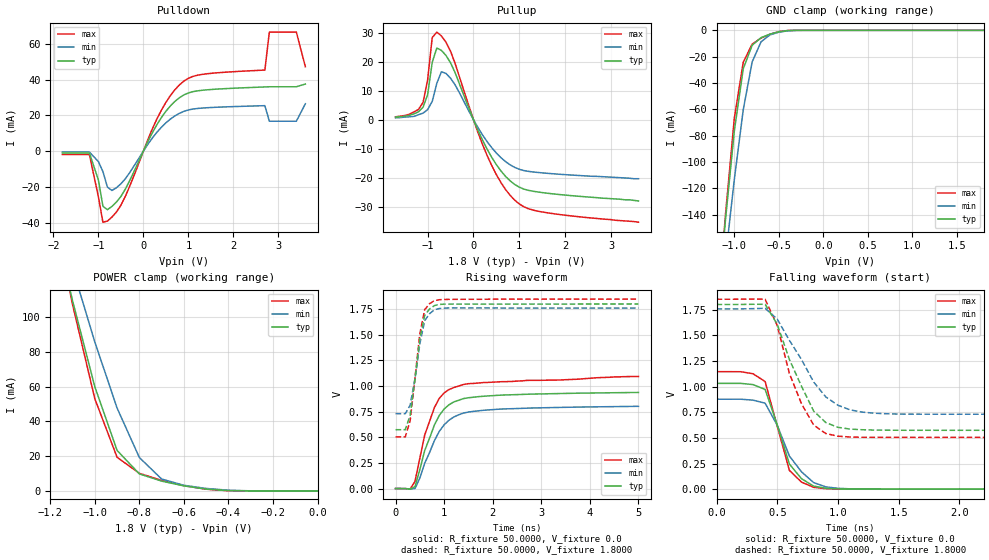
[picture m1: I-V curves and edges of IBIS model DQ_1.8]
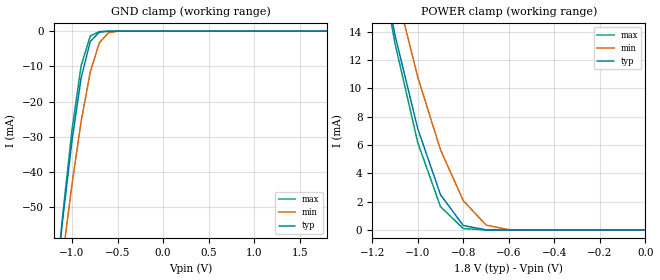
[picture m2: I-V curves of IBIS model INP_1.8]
|*** ISSI Synchronous Sram IBIS Model ***
[IBIS ver]	3.2
[File name]	is61vvps204836b100tq.ibs
[File Rev]	1.0
[Date]	May 13,2013
[Notes]
|--- Version History --------------------------------
|1.0: prelimiary
[Disclaimer]	This information is for modeling purpose only
		and is not guaranteed
[Copyright]	INTEGRATED SILICON SOLUTION, INC. 2011
[Component]	IS61VVPS204836B_100TQ
[Manufacturer]	ISSI
[Package]
| variable   typ   min   max
R_pkg		105.88m			21.330m			174.58m
L_pkg		1.8700nH		0.5900nH		2.5200nH
C_pkg		0.2100pF		0.0600pF		0.2800pF
[Pin]  signal_name   model_name   R_pin   L_pin   C_pin
100   A   INP_1.8
99   A   INP_1.8
98   CEB   INP_1.8
97   CE2   INP_1.8
96   NC   NC
95   NC   NC
94   BWbB   INP_1.8
93   BWaB   INP_1.8
92   CE2B   INP_1.8
91   VDD   POWER
90   VSS   GND
89   CLK   INP_1.8
88   GWB   INP_1.8
87   BWEB   INP_1.8
86   OEB   INP_1.8
85   ADSCB   INP_1.8
84   ADSPB   INP_1.8
83   ADVB   INP_1.8
82   A   INP_1.8
81   A   INP_1.8
80   DQPb   DQ_1.8
79   DQb   DQ_1.8
78   DQb   DQ_1.8
77   VDDQ   POWER
76   VSS   GND
75   DQb   DQ_1.8
74   DQb   DQ_1.8
73   DQb   DQ_1.8
72   DQb   DQ_1.8
71   VSS   GND
70   VDDQ   POWER
69   DQb   DQ_1.8
68   DQb   DQ_1.8
67   VSS   GND
66   NC   NC
65   VDD   POWER
64   ZZ   INP_1.8
63   DQa   DQ_1.8
62   DQa   DQ_1.8
61   VDDQ   POWER
60   VSS   GND
59   DQa   DQ_1.8
58   DQa   DQ_1.8
57   DQa   DQ_1.8
56   DQa   DQ_1.8
55   VSS   GND
54   VDDQ   POWER
53   DQa   DQ_1.8
52   DQa   DQ_1.8
51   DQPa   DQ_1.8
50   A   INP_1.8
49   A   INP_1.8
48   A   INP_1.8
47   A   INP_1.8
46   A   INP_1.8
45   A   INP_1.8
44   A   INP_1.8
43   A   INP_1.8
42   A   INP_1.8
41   VDD   POWER
40   VSS   GND
39   A   INP_1.8
38   A   INP_1.8
37   A0   INP_1.8
36   A1   INP_1.8
35   A   INP_1.8
34   A   INP_1.8
33   A   INP_1.8
32   A   INP_1.8
31   MODE   INP_1.8
30   DQPd   DQ_1.8
29   DQd   DQ_1.8
28   DQd   DQ_1.8
27   VDDQ   POWER
26   VSS   GND
25   DQd   DQ_1.8
24   DQd   DQ_1.8
23   DQd   DQ_1.8
22   DQd   DQ_1.8
21   VSS   GND
20   VDDQ   POWER
19   DQd   DQ_1.8
18   DQd   DQ_1.8
17   VSS   GND
16   NC   NC
15   VDD   POWER
14   NC   NC
13   DQc   DQ_1.8
12   DQc   DQ_1.8
11   VDDQ   POWER
10   VSS   GND
9   DQc   DQ_1.8
8   DQc   DQ_1.8
7   DQc   DQ_1.8
6   DQc   DQ_1.8
5   VSS   GND
4   VDDQ   POWER
3   DQc   DQ_1.8
2   DQc   DQ_1.8
1   DQPc   DQ_1.8
| Models and submodels in the file (2): DQ_1.8 (3-state), INP_1.8 (Input)
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|   Model DQ_1.8
[Model]		DQ_1.8
Model_type	3-state
Polarity   Non-Inverting
Enable   Active-Low
Vmeas = 	0.7500V
Cref = 		5.0000pF
Rref = 		50.0000
Vref = 		0.8000V
C_comp   3.8290pF   3.3420pF   4.0300pF|
[Temperature Range]	  25.0000   100.0000   0.0
[Voltage Range]   1.8000V   1.7000V   1.9000V
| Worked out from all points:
|   slope of the pulldown table from 0 to 0.27 V, typ, clamps not added: 20.1 ohm
|   slope of the pullup table from 0 to 0.27 V, typ, clamps not added: 29.1 ohm
|   GND clamp passes 1 mA (typ) near -0.49 V on its own axis
|   POWER clamp passes 1 mA (typ) near -0.49 V on its own axis
|   rising waveform, R_fixture 50.0000, V_fixture 0.0: 20-80 % time 458ps typ, 504ps min, 428ps max; typ from 0 V to 0.937 V
|   rising waveform, R_fixture 50.0000, V_fixture 1.8000: 20-80 % time 212ps typ, 215ps min, 202ps max; typ from 0.574 V to 1.8 V
|   falling waveform, R_fixture 50.0000, V_fixture 0.0: 20-80 % time 184ps typ, 232ps min, 159ps max; typ from 1.03 V to 0 V
|   falling waveform, R_fixture 50.0000, V_fixture 1.8000: 20-80 % time 261ps typ, 323ps min, 225ps max; typ from 1.8 V to 0.574 V
[Pulldown]
|Voltage	  I(typ)   I(min)   I(max)
-1.8V     -1.1mA     -531.4uA   -1.933mA
-1.2V     -1.1mA     -531.4uA   -1.933mA
-1V       -16.17mA   -5.85mA    -25.61mA
-900mV    -30.82mA   -11.44mA   -39.73mA
-800mV    -32.74mA   -20.11mA   -39.13mA
-400mV    -21.21mA   -15.41mA   -25.25mA
400mV     18.75mA    13.32mA    22.87mA
900mV     31.42mA    22.22mA    39.13mA
2.7V      35.87mA    25.41mA    45.31mA
2.8V      35.97mA    16.71mA    66.53mA
3.4V      35.97mA    16.71mA    66.53mA
3.6V      37.5mA     26.46mA    47.19mA
[Pullup]
|Voltage	  I(typ)   I(min)   I(max)
-1.7V     900uA      630uA      990uA
-1.3V     2mA        1.134mA    2.662mA
-1.1V     4.3mA      2.25mA     5.962mA
-1V       8.6mA      3.483mA    13.72mA
-900mV    19.73mA    6.273mA    28.28mA
-800mV    24.69mA    12.51mA    30.17mA
-700mV    23.88mA    16.48mA    28.87mA
-500mV    19.6mA     14.29mA    23.58mA
300mV     -10.22mA   -7.61mA    -12.41mA
900mV     -22.31mA   -16.43mA   -27.72mA
1.5V      -25.11mA   -18.32mA   -31.79mA
3.6V      -28mA      -20.34mA   -35.31mA
[GND_clamp]
|Voltage	  I(typ)   I(min)   I(max)
-1.8V     -699.5mA   -630.9mA   -769.6mA
-1.2V     -220.2mA   -237.3mA   -225.5mA
-1.1V     -144.4mA   -173.5mA   -140.5mA
-1V       -76.37mA   -113.2mA   -66.75mA
-900mV    -29.2mA    -60.35mA   -24.21mA
-800mV    -11.34mA   -23.99mA   -10.5mA
-700mV    -5.573mA   -8.7mA     -5.882mA
-600mV    -2.907mA   -3.456mA   -3.007mA
-500mV    -1.075mA   -1.407mA   -999.2uA
-400mV    -173.9uA   -365.4uA   -128uA
1.8V      2.34nA     184.5nA    2.08nA
[POWER_clamp]
|Voltage	  I(typ)   I(min)   I(max)
-1.8V     524.9mA    464.4mA    580.5mA
-1.2V     164.3mA    173.4mA    169.2mA
-1.1V     109.5mA    128.3mA    107.3mA
-1V       59.99mA    85.74mA    53.06mA
-900mV    23.31mA    47.72mA    19.37mA
-800mV    9.803mA    19.24mA    10.14mA
-700mV    5.64mA     6.854mA    6.056mA
-600mV    2.92mA     3.245mA    3.006mA
-500mV    1.061mA    1.426mA    981.4uA
-400mV    183.6uA    396.9uA    135.3uA
0V        2.34nA     17.95nA    3.205nA
[Ramp]
| variable   typ   min   max
dV/dt_r		0.5623/0.4256n   0.4811/0.4247n   0.6354/0.4100n
dV/dt_f		0.7357/0.2222n   0.6457/0.2069n   0.7931/0.2538n
R_load =	50.0000
[Rising Waveform]
R_fixture=	50.0000
V_fixture=	0.0
V_fixture_min=	0.0
V_fixture_max=	0.0
|time   V(typ)   V(min)   V(max)
0s        0V         0V         0V
300ps     -6.035mV   -4.762mV   -4.194mV
400ps     18.96mV    486.8uV    69.03mV
600ps     370.5mV    247mV      521.7mV
800ps     620mV      467.9mV    790.2mV
900ps     712.9mV    557.2mV    879.6mV
1.1ns     817.3mV    666.8mV    965.5mV
1.4ns     877.6mV    736.7mV    1.015V
1.9ns     903.3mV    766.6mV    1.035V
5ns       937.2mV    801.8mV    1.093V
[Rising Waveform]
R_fixture=	50.0000
V_fixture=	1.8000
V_fixture_min=	1.8500
V_fixture_max=	1.7500
|time   V(typ)   V(min)   V(max)
0s        573.8mV    730.3mV    504.1mV
200ps     573.9mV    730.3mV    504.2mV
300ps     713.7mV    812.3mV    659.4mV
400ps     1.067V     1.071V     1.076V
500ps     1.46V      1.412V     1.51V
600ps     1.689V     1.637V     1.745V
700ps     1.752V     1.705V     1.802V
800ps     1.784V     1.744V     1.833V
1.2ns     1.799V     1.762V     1.845V
5ns       1.8V       1.76V      1.848V
[Falling Waveform]
R_fixture=	50.0000
V_fixture=	0.0
V_fixture_min=	0.0
V_fixture_max=	0.0
|time   V(typ)   V(min)   V(max)
0s        1.031V     876.6mV    1.145V
300ps     1.019V     867.6mV    1.125V
400ps     972.5mV    838.1mV    1.049V
500ps     626.1mV    622.4mV    612.9mV
600ps     244.7mV    322.8mV    182.9mV
700ps     101.5mV    168.6mV    68.26mV
800ps     29.89mV    63.85mV    18.06mV
900ps     8.638mV    22.26mV    4.629mV
1.2ns     563.4uV    1.383mV    368.3uV
5ns       26.68uV    38.84uV    22.23uV
[Falling Waveform]
R_fixture=	50.0000
V_fixture=	1.8000
V_fixture_min=	1.8500
V_fixture_max=	1.7500
|time   V(typ)   V(min)   V(max)
0s        1.8V       1.757V     1.851V
400ps     1.802V     1.763V     1.851V
500ps     1.607V     1.657V     1.594V
600ps     1.264V     1.45V      1.127V
700ps     1.002V     1.263V     831.3mV
800ps     760.7mV    1.044V     624.3mV
900ps     649.1mV    898.2mV    542.1mV
1.1ns     585.4mV    772.7mV    508.4mV
1.4ns     574.7mV    734.9mV    504.6mV
5ns       573.8mV    730.3mV    504.2mV
|   Model INP_1.8
[Model]		INP_1.8
Model_type	Input
Polarity   Non-Inverting
Enable   Active-Low
Vinl = 		0.4000V
Vinh = 		1.6000V
C_comp   3.8290pF   3.3420pF   4.0300pF|
[Temperature Range]	  25.0000   100.0000   0.0
[Voltage Range]   1.8000V   1.7000V   1.9000V
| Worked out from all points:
|   GND clamp passes 1 mA (typ) near -0.73 V on its own axis
|   POWER clamp passes 1 mA (typ) near -0.83 V on its own axis
[GND_clamp]
|Voltage	  I(typ)   I(min)   I(max)
-1.8V     -237.3mA   -225.6mA   -256.2mA
-1.2V     -76.89mA   -84.89mA   -78.19mA
-1.1V     -52.83mA   -63.46mA   -51.66mA
-1V       -30.98mA   -43.42mA   -27.92mA
-900mV    -13.28mA   -25.61mA   -9.811mA
-800mV    -2.971mA   -11.61mA   -1.401mA
-700mV    -287uA     -3.303mA   -148.3uA
-600mV    -52.18uA   -480.7uA   -48.72uA
-500mV    -11.21uA   -45.78uA   -9.079uA
-400mV    -777.9nA   -4.481uA   -394.5nA
1.8V      1.69nA     1.724nA    1.796nA
[POWER_clamp]
|Voltage	  I(typ)   I(min)   I(max)
-1.8V     89.26mA    83.96mA    96.39mA
-1.2V     21.9mA     24.63mA    22.02mA
-1.1V     13.77mA    17.21mA    13.19mA
-1V       7.16mA     10.8mA     6.179mA
-900mV    2.488mA    5.659mA    1.649mA
-800mV    312.9uA    2.071mA    100.3uA
-700mV    9.014uA    348.8uA    1.66uA
-600mV    208.4nA    21.46uA    65.15nA
0V        1.69nA     1.088nA    2.855nA
